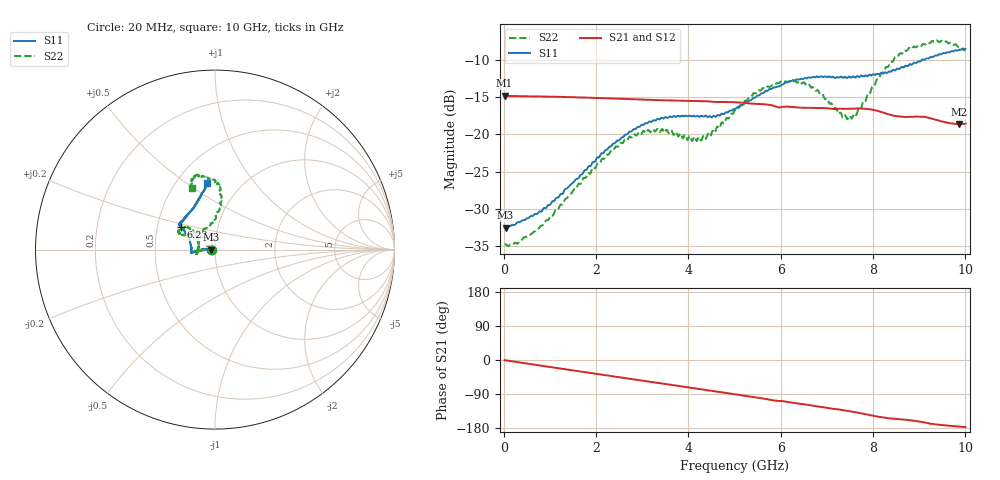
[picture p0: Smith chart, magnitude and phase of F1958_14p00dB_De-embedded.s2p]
! Integrated Device Technology
! Corporate Headquarters
! 6024 Silver Creek Valley Road
! San Jose, CA 95138  USA
! Phone:  1-408-284-8200
! Toll Free:  1-800-223-1366
! Webpage:  http://www.idt.com/
! Timing and RF Division
! 515 Groton Road, Suite 102
! Westford, MA 01886-6024
! Device:  F1958
! Description: 7-bit 0.25 dB Digital Step Attenuator
! Frequency:  0.001 -  6.000 GHz
! Package:  4x4 mm Thin QFN Plastic Package: 24 pin
! Ports:  2 RF, 12 DC
!  Pin  1  = D0
!  Pin  2  = VDD
!  Pin  3  = VMODE
!  Pin  4  = GND
!  Pin  5  = RF1  =  Port 1
!  Pin  6  = GND
!  Pin  7  = GND
!  Pin  8  = GND
!  Pin  9  = GND
!  Pin 10  = GND
!  Pin 11  = GND
!  Pin 12  = GND
!  Pin 13  = GND
!  Pin 14  = RF2  =  Port 2
!  Pin 15  = GND
!  Pin 16  = LE
!  Pin 17  = CLK
!  Pin 18  = DATA
!  Pin 19  = D6
!  Pin 20  = D5
!  Pin 21  = D4
!  Pin 22  = D3
!  Pin 23  = D2
!  Pin 24  = D1
! State:  56
! Atten State:  14.00 dB
! Voltage:  +3.30 Volts
! Current:  0.258 mA
! Data:  The device was measured on a F1958 evaluation board which has
!  individual transmission lines to the RF pins.  Data was collected
!  using a calibrated network analyzer.  The evaluation board was
!  de-embedded using Automatic Fixture Removal (AFR).
!  The reference plane is the edge of the package pin.
! Misc:
!  Action Tracker AT0419
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# GHz S dB R 50
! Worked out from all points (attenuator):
!   500 points, 20 MHz to 10 GHz, reference 50 ohm
!   highest |S21| = -14.80 dB at 20 MHz (marker M1); lowest = -18.6 dB at 9.86 GHz (marker M2)
!   lowest |S11| = -32.6 dB at 40 MHz (marker M3), VSWR 1.05, Z = 47.7 - j0.0812 ohm
!   |S11| at or under -10 dB: start of sweep to 9.053 GHz
!   |S22| runs from -35.0 to -7.3 dB; largest |S21 - S12| = 0.00052
!   S11 on the Smith chart (normalised r, x): 20 MHz: 0.95, -0.00; 6.22 GHz: 0.66, +0.17; 10 GHz: 0.70, +0.60
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0.02  -32.56 -178.0  -14.80 -0.5  -14.80 -0.5  -34.84 -177.6
0.04  -32.57 -177.9  -14.81 -0.9  -14.80 -0.8  -34.77 -176.7
0.32  -31.82 178.1  -14.85 -6.0  -14.85 -6.0  -34.58 178.6
0.72  -30.71 178.5  -14.89 -13.3  -14.88 -13.3  -32.82 -179.9
1.7  -25.37 179.3  -15.03 -31.0  -15.03 -31.0  -26.22 -179.3
2.6  -20.30 -177.2  -15.22 -47.2  -15.20 -47.2  -20.95 -174.6
2.92  -18.98 -174.5  -15.28 -52.9  -15.26 -53.0  -19.73 -171.3
3.36  -17.97 -172.4  -15.39 -60.8  -15.39 -60.9  -19.54 -166.9
4.3  -17.51 -178.6  -15.52 -77.4  -15.53 -77.5  -20.54 164.8
4.52  -17.64 175.3  -15.62 -81.5  -15.63 -81.5  -19.50 155.7
5.02  -16.56 161.5  -15.67 -90.5  -15.68 -90.5  -16.62 140.7
5.54  -14.71 151.0  -15.91 -100.1  -15.91 -100.2  -14.06 141.7
6.22  -12.84 146.8  -16.30 -112.1  -16.31 -112.1  -12.83 152.7
6.68  -12.29 144.4  -16.43 -120.1  -16.44 -120.0  -13.68 155.0
7.3  -12.21 137.9  -16.54 -131.5  -16.55 -131.4  -17.06 134.6
7.5  -12.26 135.1  -16.55 -135.3  -16.55 -135.2  -17.50 116.4
7.68  -12.22 132.1  -16.50 -139.1  -16.49 -139.1  -16.59 99.2
8.34  -11.53 116.2  -17.30 -153.8  -17.30 -153.9  -10.76 82.9
8.68  -10.88 109.5  -17.65 -157.4  -17.65 -157.4  -8.67 87.3
9.26  -9.54 101.5  -17.87 -168.2  -17.87 -168.4  -7.53 100.1
9.86  -8.60 97.1  -18.61 -175.5  -18.64 -175.3  -8.22 109.3
10  -8.50 97.1  -18.56 -177.1  -18.59 -177.1  -8.73 110.2
